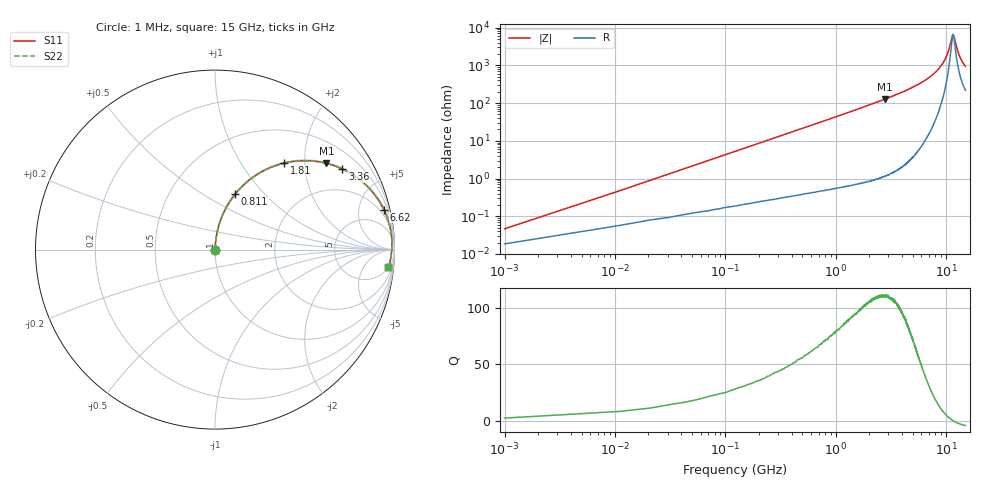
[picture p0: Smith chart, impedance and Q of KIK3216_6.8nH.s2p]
!version-2
!date-01.2022
!Series
# MHz S RI R 50
!Freq ReS11 ImS11 ReS21 ImS21 ReS12 ImS12 ReS22 ImS22
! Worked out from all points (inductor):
!   1501 points, 1 MHz to 15 GHz, reference 50 ohm
!   read as one part in series: L = 6.8 nH near 71 MHz
!   highest Q = 111 at 2.82 GHz (marker M1), where L = 7.23 nH
!   self-resonance near 11.62 GHz
!   S11 on the Smith chart (normalised r, x): 1 MHz: 1.00, +0.00; 811 MHz: 1.01, +0.70; 1.81 GHz: 1.02, +1.59; 3.36 GHz: 1.03, +3.14; 6.62 GHz: 1.22, +8.39; 15 GHz: 5, -18
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1  0.00017 0.000427  0.9998 -0.000427  0.9998 -0.000427  0.00017 0.000427
81  0.00272 0.0345  0.9973 -0.0345  0.9973 -0.0345  0.00272 0.0345
121  0.00452 0.0514  0.9955 -0.0514  0.9955 -0.0514  0.00452 0.0514
171  0.00749 0.0724  0.9925 -0.0724  0.9925 -0.0724  0.00749 0.0724
271  0.0159 0.1137  0.9841 -0.1137  0.9841 -0.1137  0.0159 0.1137
411  0.0331 0.1694  0.9669 -0.1694  0.9669 -0.1694  0.0331 0.1694
811  0.1115 0.3079  0.8885 -0.3079  0.8885 -0.3079  0.1115 0.3079
1240  0.2261 0.4126  0.7739 -0.4126  0.7739 -0.4126  0.2261 0.4126
1810  0.3872 0.4822  0.6128 -0.4822  0.6128 -0.4822  0.3872 0.4822
2510  0.5584 0.4921  0.4416 -0.4921  0.4416 -0.4921  0.5584 0.4921
2820  0.6204 0.4808  0.3796 -0.4808  0.3796 -0.4808  0.6204 0.4808
3360  0.709 0.4495  0.291 -0.4495  0.291 -0.4495  0.709 0.4495
5010  0.8705 0.3289  0.1295 -0.3289  0.1295 -0.3289  0.8705 0.3289
6620  0.9409 0.2228  0.0591 -0.2228  0.0591 -0.2228  0.9409 0.2228
7510  0.9615 0.1727  0.0385 -0.1727  0.0385 -0.1727  0.9615 0.1727
8940  0.9795 0.1032  0.0205 -0.1032  0.0205 -0.1032  0.9795 0.1032
10010  0.985 0.0584  0.015 -0.0584  0.015 -0.0584  0.985 0.0584
11540  0.9852 0.00259  0.0148 -0.00259  0.0148 -0.00259  0.9852 0.00259
11790  0.9846 -0.00575  0.0154 0.00575  0.0154 0.00575  0.9846 -0.00575
12510  0.982 -0.0286  0.018 0.0286  0.018 0.0286  0.982 -0.0286
13550  0.9766 -0.0592  0.0234 0.0592  0.0234 0.0592  0.9766 -0.0592
15000  0.9662 -0.0973  0.0338 0.0973  0.0338 0.0973  0.9662 -0.0973
